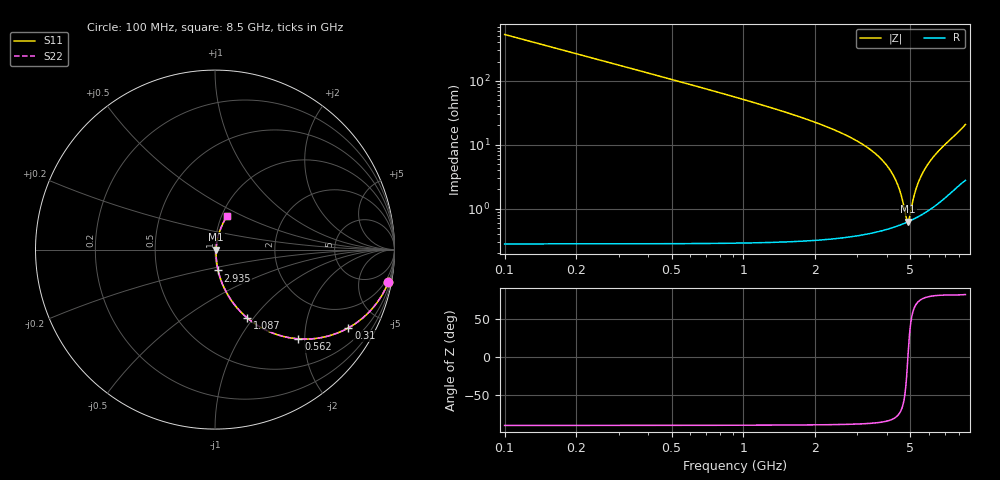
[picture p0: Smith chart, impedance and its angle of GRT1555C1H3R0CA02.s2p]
!Murata Part Number: GRT1555C1H3R0CA02
!These Parameters are Measured in Series Mode Connection
!Data Generated on Jun 19, 2026
!  o--ll--o
!Port1  Port2
!  o------o
!Operation Temp=25[degC], DC Bias Voltage=0[V]
!Freq. Start=100[MHz] Stop=9[GHz] 401[Steps]
# Hz S RI R 50
!Freq.(Hz) S11(Real) S11(Imag) S21(Real) S21(Imag) S12(Real) S12(Imag) S22(Real) S22(Imag)
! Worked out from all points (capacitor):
!   401 points, 100 MHz to 8.5 GHz, reference 50 ohm
!   read as one part in series: C = 3 pF near 142 MHz
!   lowest |Z| = 623 mohm at 4.888 GHz (marker M1)
!   series resonance near 4.884 GHz, so ESL is about 350 pH
!   S11 on the Smith chart (normalised r, x): 100 MHz: 1, -11; 310 MHz: 1.01, -3.41; 562 MHz: 1.01, -1.86; 1.087 GHz: 1.01, -0.93; 2.935 GHz: 1.01, -0.24; 8.5 GHz: 1.06, +0.41
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1e8  0.9656 -0.1821  0.0344 0.1821  0.0344 0.1821  0.9656 -0.1821
2.05e8  0.8694 -0.3364  0.1306 0.3364  0.1306 0.3364  0.8694 -0.3364
3.1e8  0.7437 -0.4358  0.2563 0.4358  0.2563 0.4358  0.7437 -0.4358
4.15e8  0.617 -0.485  0.383 0.485  0.383 0.485  0.617 -0.485
5.62e8  0.4652 -0.4973  0.5348 0.4973  0.5348 0.4973  0.4652 -0.4973
7.93e8  0.2995 -0.4559  0.7005 0.4559  0.7005 0.4559  0.2995 -0.4559
1.087e9  0.1797 -0.3808  0.8203 0.3808  0.8203 0.3808  0.1797 -0.3808
1.507e9  0.0955 -0.2893  0.9045 0.2893  0.9045 0.2893  0.0955 -0.2893
2.914e9  0.0179 -0.118  0.9821 0.118  0.9821 0.118  0.0179 -0.118
2.935e9  0.0175 -0.1163  0.9825 0.1163  0.9825 0.1163  0.0175 -0.1163
3.754e9  0.00805 -0.06  0.9919 0.06  0.9919 0.06  0.00805 -0.06
4.3e9  0.006 -0.0293  0.994 0.0293  0.994 0.0293  0.006 -0.0293
4.531e9  0.00581 -0.0174  0.9942 0.0174  0.9942 0.0174  0.00581 -0.0174
4.804e9  0.00603 -0.00384  0.994 0.00384  0.994 0.00384  0.00603 -0.00384
4.888e9  0.00618 0.000215  0.9938 -0.000215  0.9938 -0.000215  0.00618 0.000215
4.951e9  0.00633 0.00323  0.9937 -0.00323  0.9937 -0.00323  0.00633 0.00323
5.14e9  0.0069 0.0121  0.9931 -0.0121  0.9931 -0.0121  0.0069 0.0121
5.287e9  0.00748 0.019  0.9925 -0.019  0.9925 -0.019  0.00748 0.019
5.707e9  0.00981 0.0381  0.9902 -0.0381  0.9902 -0.0381  0.00981 0.0381
6.295e9  0.0149 0.0644  0.9851 -0.0644  0.9851 -0.0644  0.0149 0.0644
7.114e9  0.026 0.1021  0.974 -0.1021  0.974 -0.1021  0.026 0.1021
8.5e9  0.0642 0.1868  0.9358 -0.1868  0.9358 -0.1868  0.0642 0.1868
